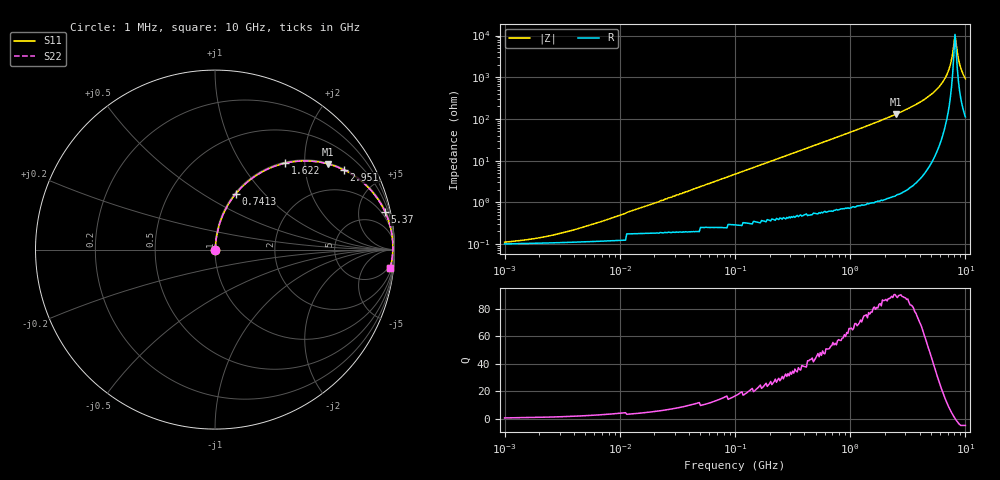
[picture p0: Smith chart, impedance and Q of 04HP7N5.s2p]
# MHz S MA R 50
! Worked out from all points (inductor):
!   401 points, 1 MHz to 10 GHz, reference 50 ohm
!   read as one part in series: L = 7.5 nH near 7.586 MHz
!   highest Q = 89.5 at 2.512 GHz (marker M1), where L = 8.29 nH
!   self-resonance near 8.128 GHz
!   S11 on the Smith chart (normalised r, x): 1 MHz: 1.00, +0.00; 741.3 MHz: 1.01, +0.70; 1.622 GHz: 1.02, +1.59; 2.951 GHz: 1.04, +3.20; 5.37 GHz: 1.22, +8.96; 10 GHz: 3, -18
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1  0.001108 25.1  0.999 -0.0  0.999 -0.0  0.001108 25.1
2.138  0.001489 42.5  0.999 -0.1  0.999 -0.1  0.001489 42.5
4.677  0.002526 60.5  0.999 -0.1  0.999 -0.1  0.002526 60.5
21.878  0.01 79.8  0.998 -0.6  0.998 -0.6  0.01 79.8
102.329  0.048 83.8  0.996 -2.8  0.996 -2.8  0.048 83.8
467.735  0.215 76.2  0.972 -12.4  0.972 -12.4  0.215 76.2
741.31  0.33 69.7  0.938 -19.3  0.938 -19.3  0.33 69.7
1621.81  0.619 51.0  0.778 -38.2  0.778 -38.2  0.619 51.0
2187.762  0.739 41.7  0.665 -47.7  0.665 -47.7  0.739 41.7
2511.886  0.79 37.2  0.604 -52.2  0.604 -52.2  0.79 37.2
2951.209  0.844 31.8  0.527 -57.5  0.527 -57.5  0.844 31.8
4168.694  0.932 20.5  0.35 -68.7  0.35 -68.7  0.932 20.5
5370.318  0.971 12.5  0.217 -76.0  0.217 -76.0  0.971 12.5
6165.95  0.983 8.3  0.144 -79.1  0.144 -79.1  0.983 8.3
6918.31  0.989 4.8  0.085 -80.1  0.085 -80.1  0.989 4.8
7413.102  0.991 2.8  0.049 -77.7  0.049 -77.7  0.991 2.8
7943.282  0.991 0.7  0.016 -54.1  0.016 -54.1  0.991 0.7
8128.305  0.991 0.0  0.009338 -5.2  0.009338 -5.2  0.991 0.0
8511.38  0.99 -1.3  0.025 65.1  0.025 65.1  0.99 -1.3
9120.108  0.987 -3.4  0.06 75.8  0.06 75.8  0.987 -3.4
9549.926  0.985 -4.7  0.083 77.0  0.083 77.0  0.985 -4.7
10000  0.981 -6.1  0.107 76.9  0.107 76.9  0.981 -6.1
